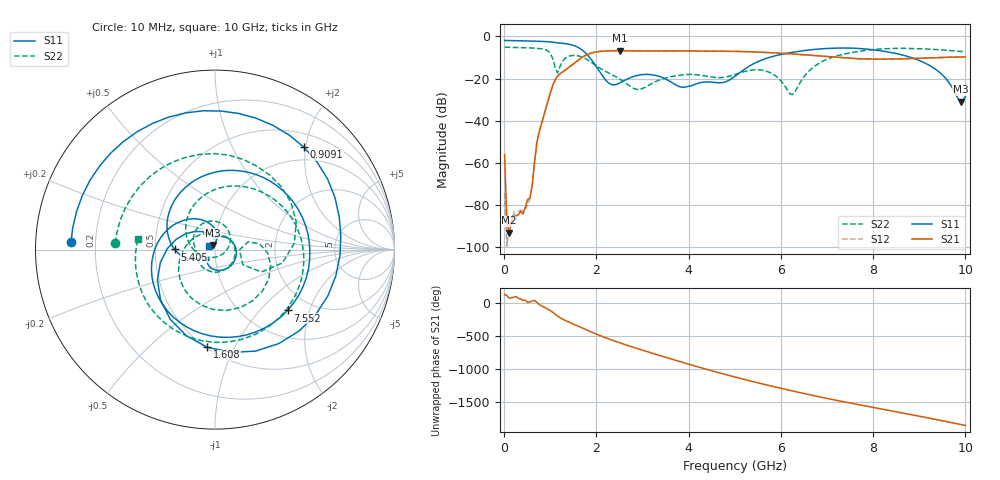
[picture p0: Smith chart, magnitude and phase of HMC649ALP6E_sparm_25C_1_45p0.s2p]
!Analog Devices Inc..
!GaAs MMIC 6-BIT DIGITAL PHASE SHIFTER, 3 - 6 GHz
!Filename: HMC649ALP6E_sparm_25C_1_45p0.s2p
!  :25C = 25degC
!  :_1_ = Sn1
!  :_45p0  = 45.0 state
!Device type:
!2 Port Calibration to sma connectors
!Phase Shifter:  0.000
!	Vss= -5V, Vdd= +5V , control Voltage = 0/ +5V
!Freq	S11	S11	S21	S21	S12	S12	S22	S22
! GHz	Mag dB	Degrees	Mag dB	Degrees	Mag dB	Degrees	Mag dB	Degrees
# GHZ S DB R 50.0
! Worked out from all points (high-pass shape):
!   201 points, 10 MHz to 10 GHz, reference 50 ohm
!   highest |S21| = -6.75 dB at 2.507 GHz (marker M1); lowest = -93.1 dB at 109.9 MHz (marker M2)
!   |S21| within 3 dB of the highest: 1.703 GHz to 7.128 GHz (5.425 GHz wide, 123 % of centre); 9.888 GHz to end of sweep
!   lowest |S11| = -30.9 dB at 9.9 GHz (marker M3), VSWR 1.06, Z = 48.7 + j2.51 ohm
!   |S11| at or under -10 dB: 1.854 GHz to 5.742 GHz (3.887 GHz wide, 102 % of centre); 8.825 GHz to end of sweep
!   |S22| runs from -27.6 to -5.1 dB; largest |S21 - S12| = 0.0017
!   S11 on the Smith chart (normalised r, x): 10 MHz: 0.11, +0.03; 909.1 MHz: 0.74, +1.97; 1.608 GHz: 0.51, -0.79; 5.405 GHz: 0.63, +0.00; 7.552 GHz: 1.54, -1.44; 10 GHz: 0.94, +0.04
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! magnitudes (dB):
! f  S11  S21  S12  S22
! 10 MHz  -1.9  -56.2  -74.3  -5.1
! 59.95 MHz  -1.9  -88.1  -99.5  -5.1
! 109.9 MHz  -1.9  -93.1  -88.2  -5.1
! 509.5 MHz  -2.1  -77.4  -80.2  -5.4
! 609.4 MHz  -2.2  -70.5  -70.3  -5.5
! 709.3 MHz  -2.3  -50.4  -50.4  -5.7
! 909.1 MHz  -2.4  -33.8  -33.7  -6.4
! 1.159 GHz  -3.0  -18.8  -18.8  -17.3
! 1.608 GHz  -5.3  -11.2  -11.2  -9.2
! 1.708 GHz  -6.7  -9.7  -9.7  -9.9
! 2.507 GHz  -22.1  -6.8  -6.7  -20.2
! 3.357 GHz  -18.9  -6.9  -6.9  -20.7
! 3.906 GHz  -24.1  -6.9  -6.9  -18.2
! 5.005 GHz  -18.9  -7.1  -7.1  -18.0
! 5.405 GHz  -13.0  -7.3  -7.3  -15.9
! 6.254 GHz  -7.5  -8.3  -8.3  -27.6
! 6.703 GHz  -6.2  -9.0  -9.0  -14.6
! 7.552 GHz  -5.6  -10.4  -10.4  -7.6
! 8.352 GHz  -7.5  -10.7  -10.7  -5.7
! 9.351 GHz  -15.5  -10.1  -10.1  -6.2
! 9.9 GHz  -30.9  -9.7  -9.7  -7.1
! 10 GHz  -28.5  -9.7  -9.7  -7.3
